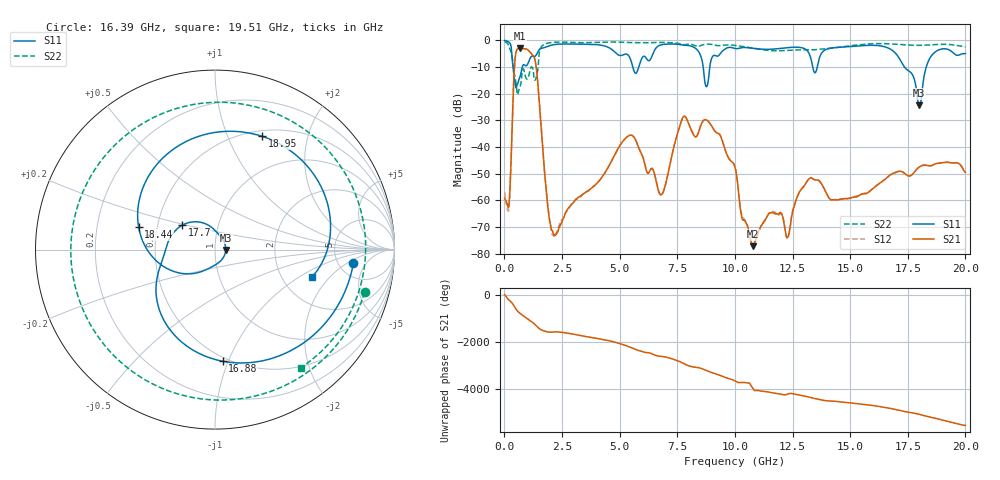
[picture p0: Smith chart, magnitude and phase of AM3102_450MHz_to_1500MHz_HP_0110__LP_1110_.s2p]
!Agilent Technologies,E8364B,MY43040894,A.07.50.67
!Agilent E8364B: A.07.50.67
!Date: Thursday, January 11, 2018 05:50:01
!Correction: S11(Full 2 Port(1,2))
!S21(Full 2 Port(1,2))
!S12(Full 2 Port(1,2))
!S22(Full 2 Port(1,2))
!S2P File: Measurements: S11, S21, S12, S22:
# Hz S  dB  R 50
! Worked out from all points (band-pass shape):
!   1601 points, 10 MHz to 20 GHz, reference 50 ohm
!   highest |S21| = -2.91 dB at 672.2 MHz (marker M1); lowest = -77.2 dB at 10.78 GHz (marker M2)
!   |S21| within 3 dB of the highest: 477.3 MHz to 1.26 GHz (782.5 MHz wide, 90.1 % of centre)
!   lowest |S11| = -24.5 dB at 18 GHz (marker M3), VSWR 1.13, Z = 56.4 - j0.213 ohm
!   |S11| at or under -10 dB: 371.9 MHz to 776.7 MHz (404.7 MHz wide, 70.5 % of centre); 8.625 GHz to 8.911 GHz (286 MHz wide, 3.26 % of centre); 17.35 GHz to 18.3 GHz (948.8 MHz wide, 5.32 % of centre)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
!   |S22| runs from -20.4 to -0.5 dB; largest |S21 - S12| = 0.0013
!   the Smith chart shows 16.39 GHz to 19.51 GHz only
!   S11 on the Smith chart (normalised r, x): 16.39 GHz: 6.94, -2.54; 16.88 GHz: 0.47, -0.95; 17.7 GHz: 0.67, +0.19; 18.44 GHz: 0.39, +0.12; 18.95 GHz: 0.56, +1.34; 19.51 GHz: 2.91, -1.31
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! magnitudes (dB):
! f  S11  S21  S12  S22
! 10 MHz  -0.1  -59.2  -56.9  -0.5
! 184.9 MHz  -0.6  -62.7  -64.0  -2.0
! 459.8 MHz  -15.9  -7.4  -7.4  -13.7
! 672.2 MHz  -13.8  -2.9  -2.9  -17.7
! 1.347 GHz  -5.9  -8.2  -8.2  -14.8
! 2.096 GHz  -1.7  -71.8  -73.1  -0.8
! 3.346 GHz  -1.5  -58.2  -58.3  -0.9
! 5.47 GHz  -7.1  -35.6  -35.6  -0.9
! 6.682 GHz  -2.1  -56.5  -56.3  -0.8
! 7.794 GHz  -1.8  -28.5  -28.5  -1.7
! 10.01 GHz  -3.1  -47.6  -47.6  -1.9
! 10.78 GHz  -3.0  -77.2  -76.9  -3.0
! 13.34 GHz  -8.5  -51.7  -51.6  -3.6
! 16.39 GHz  -2.2  -53.0  -52.9  -1.2
! 16.68 GHz  -3.0  -50.9  -51.0  -1.3
! 16.88 GHz  -4.1  -49.9  -50.0  -1.4
! 17.7 GHz  -12.9  -50.3  -50.3  -1.9
! 18 GHz  -24.5  -47.5  -47.5  -1.9
! 18.44 GHz  -7.0  -47.1  -47.1  -1.8
! 18.95 GHz  -3.3  -46.0  -46.0  -1.5
! 19.51 GHz  -5.0  -46.0  -46.0  -1.8
! 20 GHz  -5.0  -49.6  -49.3  -2.5
